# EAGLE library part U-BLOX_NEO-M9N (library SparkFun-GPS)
u-blox NEO-M9N GPS Module The NEO-M9N module is built on the robust u-blox M9 GNSS chip, which provides exceptional sensitivity and acquisition times for all L1 GNSS systems. The u-blox M9 standard precision GNSS platform, which delivers meter-level accuracy, succeeds the well-known u-blox M8 product range. The receiver also provides higher navigation rate and improved security features compared to previous u-blox GNSS generations. The NEO-M9N module is available in the NEO form factor LLC package
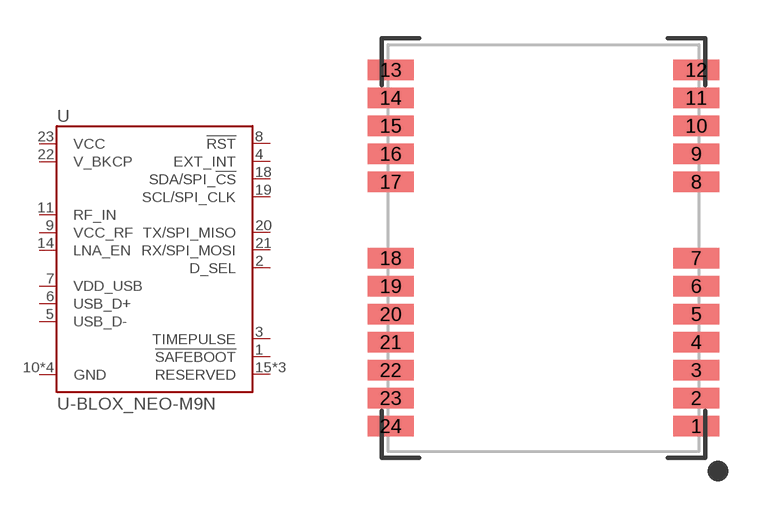
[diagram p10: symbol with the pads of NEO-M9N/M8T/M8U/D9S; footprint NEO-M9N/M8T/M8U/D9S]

Designator prefix U

## U-BLOX_NEO-M9N (PROD_ID: IC-14651)  [NEO-M9N/M8T/M8U/D9S]
1  !SAFEBOOT!
2  D_SEL
3  TIMEPULSE
4  EXT_INT
5  USB_D-
6  USB_D+
7  VDD_USB
8  !RST
9  VCC_RF
10  GND
11  RF_IN
12  GND
13  GND
14  LNA_EN
15  RESERVED  nc
16  RESERVED  nc
17  RESERVED  nc
18  SDA/SPI_!CS!
19  SCL/SPI_CLK
20  TX/SPI_MISO
21  RX/SPI_MOSI
22  V_BKCP
23  VCC
24  GND

## Footprint NEO-M9N/M8T/M8U/D9S (pad centres in mm)
u-blox NEO-M9N/M8T/M8U/D9S Module Mechanical Specifications Overall: 12.2mm x 16.0mm Pad Pitch: 1.1mm Pad Width: .8mm Pad Length: .9mm Number of Pins: 24
smd 1.8 x 0.8: 1 6,-7; 2 6,-5.9; 3 6,-4.8; 4 6,-3.7; 5 6,-2.6; 6 6,-1.5; 7 6,-0.4; 8 6,2.6; 9 6,3.7; 10 6,4.8; 11 6,5.9; 12 6,7; 13 -6,7; 14 -6,5.9; 15 -6,4.8; 16 -6,3.7; 17 -6,2.6; 18 -6,-0.4; 19 -6,-1.5; 20 -6,-2.6; 21 -6,-3.7; 22 -6,-4.8; 23 -6,-5.9; 24 -6,-7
